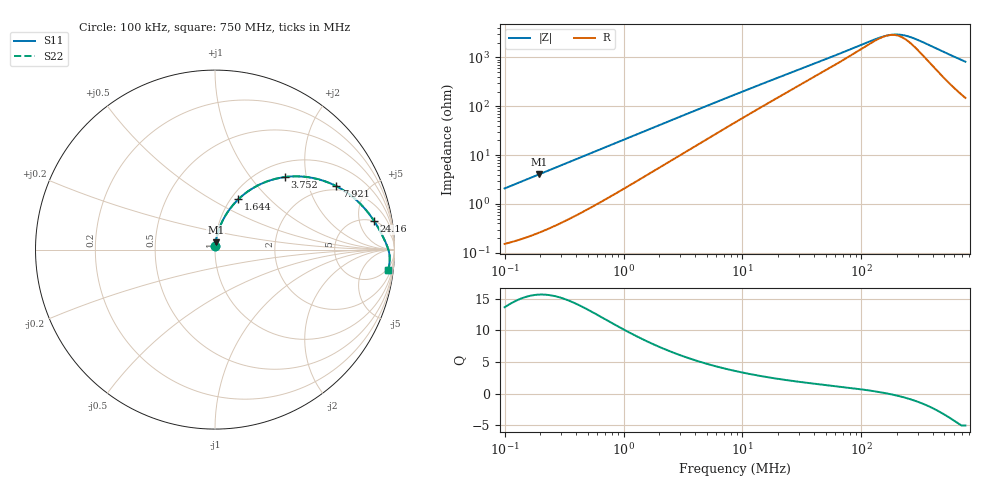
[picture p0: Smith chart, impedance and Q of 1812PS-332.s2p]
# MHz S MA R 50
!Freq  MagS11  AngS11  MagS21  AngS21  MagS12  AngS12  MagS22  AngS22
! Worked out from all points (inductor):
!   801 points, 100 kHz to 750 MHz, reference 50 ohm
!   read as one part in series: L = 3.3 uH near 104.6 kHz
!   highest Q = 15.6 at 195.3 kHz (marker M1), where L = 3.29 uH
!   self-resonance near 168.6 MHz
!   S11 on the Smith chart (normalised r, x): 100 kHz: 1.00, +0.04; 1.644 MHz: 1.08, +0.67; 3.752 MHz: 1.28, +1.51; 7.921 MHz: 1.82, +3.07; 24.16 MHz: 4.96, +8.36; 750 MHz: 4, -16
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0.1  0.02074 84.6  0.9983 -1.2  0.9983 -1.2  0.02074 84.6
0.1952673  0.04036 84.0  0.9966 -2.3  0.9966 -2.3  0.04036 84.0
0.4457309  0.0913 80.6  0.9892 -5.2  0.9892 -5.2  0.0913 80.6
0.9410423  0.1875 73.8  0.9645 -10.8  0.9645 -10.8  0.1875 73.8
1.257618  0.2447 69.7  0.9434 -14.1  0.9434 -14.1  0.2447 69.7
1.643616  0.3093 65.1  0.9138 -17.9  0.9138 -17.9  0.3093 65.1
1.964725  0.3584 61.5  0.887 -20.8  0.887 -20.8  0.3584 61.5
2.655125  0.45 54.8  0.8266 -26.4  0.8266 -26.4  0.45 54.8
3.751834  0.561 46.1  0.7326 -33.5  0.7326 -33.5  0.561 46.1
5.361003  0.6682 36.9  0.6145 -40.7  0.6145 -40.7  0.6682 36.9
7.921  0.7628 27.6  0.4794 -47.5  0.4794 -47.5  0.7628 27.6
8.660254  0.7805 25.7  0.4499 -48.7  0.4499 -48.7  0.7805 25.7
13.83475  0.8514 17.1  0.3126 -53.4  0.3126 -53.4  0.8514 17.1
24.16366  0.901 10.1  0.1948 -54.5  0.1948 -54.5  0.901 10.1
38.60143  0.9262 6.3  0.1289 -52.0  0.1289 -52.0  0.9262 6.3
128.7469  0.9612 0.9  0.04148 -20.4  0.04148 -20.4  0.9612 0.9
170.1501  0.9661 -0.0  0.03395 0.8  0.03395 0.8  0.9661 -0.0
210.3125  0.9691 -0.7  0.03319 21.1  0.03319 21.1  0.9691 -0.7
259.9547  0.9716 -1.4  0.03745 40.1  0.03745 40.1  0.9716 -1.4
310.7413  0.9733 -2.1  0.04458 52.2  0.04458 52.2  0.9733 -2.1
580.3009  0.9745 -5.0  0.09036 71.1  0.09036 71.1  0.9745 -5.0
750  0.9715 -6.7  0.1191 72.8  0.1191 72.8  0.9715 -6.7
